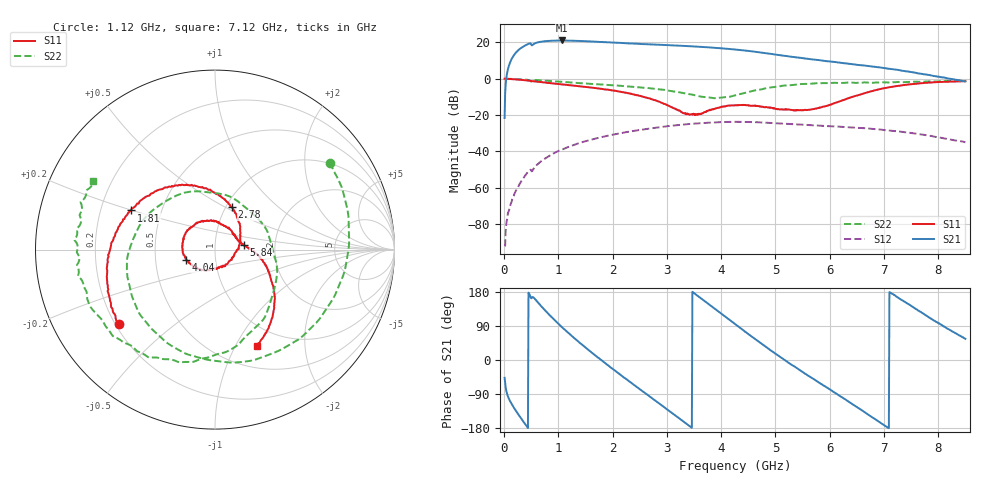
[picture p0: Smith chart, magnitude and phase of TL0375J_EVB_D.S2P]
!Agilent Technologies,E5071C,MY46523237,B.13.01
!Date: Mon Aug 08 13:48:09 2022
!Data & Calibration Information:
!Freq	S11:SOLT2(ON)	S21:SOLT2(ON)	S12:SOLT2(ON)	S22:SOLT2(ON)
!PortZ  Port1:50+j0  Port2:50+j0
!Above PortZ is port z conversion or system Z0 setting when saving the data.
!When reading, reference impedance value at option line is always used.
# Hz S dB R 50
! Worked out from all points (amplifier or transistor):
!   850 points, 10 MHz to 8.5 GHz, reference 50 ohm
!   highest |S21| = 21.0 dB at 1.06 GHz (marker M1)
!   |S21| within 3 dB of that: 371.8 MHz to 3.313 GHz (2.941 GHz wide, 160 % of centre)
!   unconditionally stable (mu >= 1): 11.54 MHz to end of sweep
!   at 1.42 GHz: K = 1.14, MAG = 25.6 dB, |S12| = -35.2 dB
!   at 4.26 GHz: K = 1.20, MAG = 17.2 dB, |S12| = -23.8 dB
!   at 8.5 GHz: K = 2.57, MAG = 9.8 dB, |S12| = -35.1 dB
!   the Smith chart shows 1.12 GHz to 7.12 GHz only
!   S11 on the Smith chart (normalised r, x): 1.12 GHz: 0.21, -0.33; 1.81 GHz: 0.33, +0.20; 2.78 GHz: 1.07, +0.54; 4.04 GHz: 0.72, -0.08; 5.84 GHz: 1.38, +0.07; 7.12 GHz: 0.75, -1.23
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1e7  -0.10 -2.1  -21.68 -47.0  -92.22 160.4  0.00 -73.7
2.4e8  -0.51 -36.9  14.93 -138.3  -60.55 116.7  -0.30 153.5
4.5e8  -1.15 -66.5  19.12 177.8  -51.00 100.2  -0.80 121.3
7.2e8  -2.07 -99.7  20.44 136.7  -44.66 82.0  -1.05 88.1
8.8e8  -2.59 -117.4  20.80 112.7  -41.73 66.9  -1.39 67.0
1.06e9  -3.18 -136.2  20.97 87.6  -39.13 48.8  -1.81 44.5
1.12e9  -3.38 -142.5  20.91 80.1  -38.41 44.2  -1.93 37.2
1.43e9  -4.34 -171.7  20.66 41.1  -35.08 15.0  -2.58 -0.4
1.81e9  -5.73 155.1  20.12 -2.5  -32.11 -20.1  -3.28 -45.1
2.31e9  -8.16 112.8  19.33 -56.7  -29.19 -66.7  -4.38 -102.5
2.78e9  -11.92 68.5  18.70 -106.6  -27.10 -109.9  -5.68 -155.5
2.84e9  -12.50 62.2  18.62 -112.8  -26.87 -115.5  -5.83 -162.8
3.14e9  -16.45 21.4  18.19 -144.8  -25.79 -143.8  -7.14 161.5
3.42e9  -19.90 -40.9  17.79 -174.8  -24.97 -170.8  -8.65 125.2
4.04e9  -15.30 -161.1  16.58 118.3  -23.91 128.4  -10.30 23.7
4.26e9  -14.64 168.3  15.98 94.4  -23.80 106.5  -9.15 -12.0
4.9e9  -15.87 90.7  13.67 26.5  -24.33 45.2  -4.93 -81.9
5.67e9  -16.94 18.3  10.57 -47.2  -25.72 -21.6  -2.78 -134.8
5.84e9  -15.83 8.6  9.96 -63.0  -25.97 -36.1  -2.57 -144.2
7.09e9  -4.82 -64.4  5.40 -179.9  -28.61 -141.4  -2.21 153.2
7.12e9  -4.66 -66.5  5.25 177.4  -28.71 -143.6  -2.19 150.7
8.5e9  -1.41 -151.5  -1.55 55.8  -35.09 109.3  -1.29 58.5
